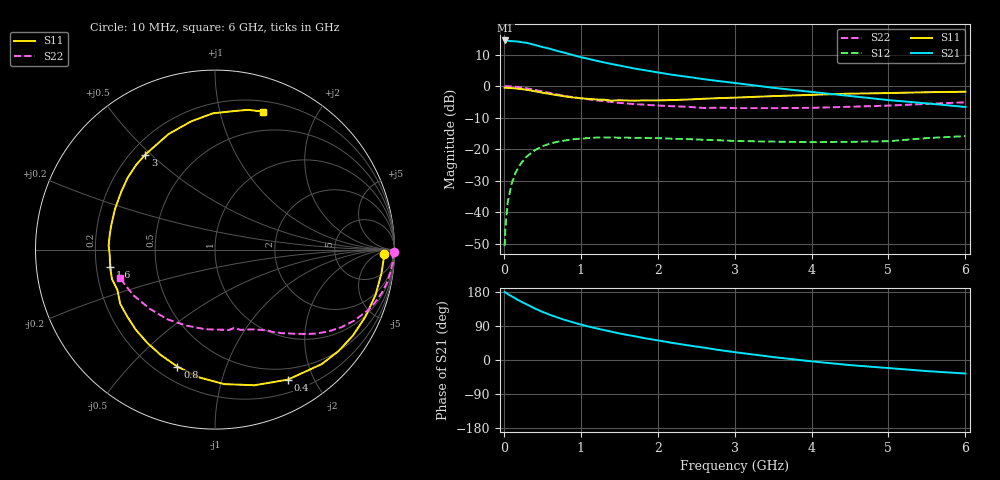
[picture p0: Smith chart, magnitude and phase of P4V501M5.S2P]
! SIEMENS Small Signal Semiconductors
! BFP182
! Si NPN RF Bipolar Junction Transistor in SOT143
! VCE = 0.5 V  IC = 1.5 mA
! Common Emitter S-Parameters:  March  1996
# GHz  S  MA  R  50
!  f  S11  S21  S12  S22
! GHz  MAG  ANG  MAG  ANG  MAG  ANG  MAG  ANG
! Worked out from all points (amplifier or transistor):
!   36 points, 10 MHz to 6 GHz, reference 50 ohm
!   highest |S21| = 14.5 dB at 20 MHz (marker M1)
!   |S21| within 3 dB of that: start of sweep to 650.5 MHz
!   unconditionally stable (mu >= 1): 2.156 GHz to end of sweep
!   at 250 MHz: K = 0.13, MSG = 18.8 dB, |S12| = -23.7 dB
!   at 1.4 GHz: K = 0.67, MSG = 11.6 dB, |S12| = -16.3 dB
!   at 6 GHz: K = 1.35, MAG = 1.1 dB, |S12| = -15.9 dB
!   S11 on the Smith chart (normalised r, x): 10 MHz: 28, -13; 400 MHz: 0.35, -1.65; 800 MHz: 0.28, -0.69; 1.6 GHz: 0.26, -0.08; 3 GHz: 0.26, +0.48; 6 GHz: 0.30, +1.37
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0.01  0.9428 -1.6  5.215 179.3  0.0029 86.2  0.9957 -0.7
0.02  0.941 -3.3  5.293 178.4  0.0056 85.8  0.9903 -1.5
0.05  0.9368 -8.1  5.243 174.2  0.0142 86.0  0.9935 -3.8
0.1  0.9296 -15.8  5.157 168.4  0.0279 79.4  0.9853 -7.5
0.15  0.9171 -24.4  5.132 162.4  0.0418 75.1  0.9745 -11.2
0.25  0.8908 -39.4  4.929 151.4  0.0655 66.0  0.9402 -18.1
0.3  0.8721 -47.0  4.844 146.6  0.0769 61.8  0.9193 -21.3
0.4  0.8305 -60.7  4.506 136.2  0.0957 53.9  0.8723 -26.9
0.5  0.787 -73.8  4.167 127.2  0.111 46.7  0.826 -31.6
0.6  0.7512 -86.1  3.91 119.2  0.1229 40.5  0.7791 -35.8
0.7  0.7165 -97.6  3.594 112.0  0.1311 35.2  0.7369 -39.3
0.8  0.6849 -107.8  3.353 105.3  0.1376 30.6  0.6991 -42.3
0.9  0.6606 -117.1  3.101 99.4  0.1435 26.5  0.6675 -44.7
1.1  0.6272 -134.9  2.706 88.3  0.1501 19.6  0.6163 -49.2
1.3  0.6085 -150.3  2.379 79.1  0.1532 13.7  0.5766 -53.1
1.6  0.592 -170.5  2.008 66.3  0.1524 7.6  0.5309 -58.0
2.2  0.6014 157.9  1.506 44.8  0.1463 -0.4  0.4794 -68.3
3  0.6565 126.3  1.122 20.7  0.1353 -4.9  0.4481 -85.0
3.5  0.6935 112.0  0.94 7.8  0.1318 -4.9  0.4472 -96.9
4.5  0.7594 90.9  0.697 -13.5  0.1307 -2.1  0.4705 -124.4
5.5  0.7999 76.8  0.532 -29.3  0.1498 2.1  0.5227 -151.2
6  0.8144 70.7  0.467 -35.7  0.1612 0.5  0.5531 -163.5
